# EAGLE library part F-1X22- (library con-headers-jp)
FEMALE HEADER
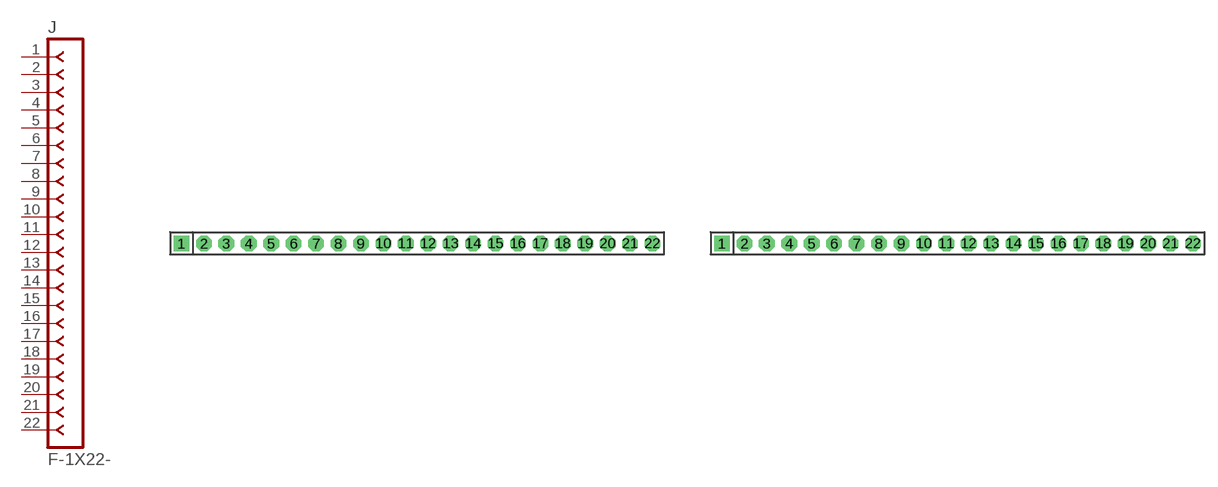
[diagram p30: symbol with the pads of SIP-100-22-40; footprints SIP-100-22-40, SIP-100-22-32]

Designator prefix J

## F-1X22-SIP-100-40  [SIP-100-22-40]
1  1  pas
2  2  pas
3  3  pas
4  4  pas
5  5  pas
6  6  pas
7  7  pas
8  8  pas
9  9  pas
10  10  pas
11  11  pas
12  12  pas
13  13  pas
14  14  pas
15  15  pas
16  16  pas
17  17  pas
18  18  pas
19  19  pas
20  20  pas
21  21  pas
22  22  pas

## F-1X22-SIP-100-32  [SIP-100-22-32]
Pads as for SIP-100-22-40

## F-1X22-SIP-100-32Y  [SIP-100-22-32Y]
Pads as for SIP-100-22-40

## F-1X22-SIP-100-40Y  [SIP-100-22-40Y]
Pads as for SIP-100-22-40

## F-1X22-KK-4455-B22  [KK-4455-B22]
Pads as for SIP-100-22-40

## F-1X22-KK-4455-C22  [KK-4455-C22]
Pads as for SIP-100-22-40

## F-1X22-KK-4455-A22  [KK-4455-A22]
Pads as for SIP-100-22-40

## Footprint SIP-100-22-40 (pad centres in mm)
SIP Header - 0.1", 40 mil drill
drill 1.016 pad 1.778 square: 1 -26.67,0
drill 1.016 pad 1.778 octagon: 2 -24.13,0; 3 -21.59,0; 4 -19.05,0; 5 -16.51,0; 6 -13.97,0; 7 -11.43,0; 8 -8.89,0; 9 -6.35,0; 10 -3.81,0; 11 -1.27,0; 12 1.27,0; 13 3.81,0; 14 6.35,0; 15 8.89,0; 16 11.43,0; 17 13.97,0; 18 16.51,0; 19 19.05,0; 20 21.59,0; 21 24.13,0; 22 26.67,0

## Footprint SIP-100-22-32 (pad centres in mm)
SIP Header - 0.1", 32 mil drill
drill 0.813 pad 1.778 square: 1 -26.67,0
drill 0.813 pad 1.778 octagon: 2 -24.13,0; 3 -21.59,0; 4 -19.05,0; 5 -16.51,0; 6 -13.97,0; 7 -11.43,0; 8 -8.89,0; 9 -6.35,0; 10 -3.81,0; 11 -1.27,0; 12 1.27,0; 13 3.81,0; 14 6.35,0; 15 8.89,0; 16 11.43,0; 17 13.97,0; 18 16.51,0; 19 19.05,0; 20 21.59,0; 21 24.13,0; 22 26.67,0

## Footprint SIP-100-22-32Y (pad centres in mm)
SIP Header - 0.1", 32 mil drill
drill 0.813 long: 1 -26.67,0; 2 -24.13,0; 3 -21.59,0; 4 -19.05,0; 5 -16.51,0; 6 -13.97,0; 7 -11.43,0; 8 -8.89,0; 9 -6.35,0; 10 -3.81,0; 11 -1.27,0; 12 1.27,0; 13 3.81,0; 14 6.35,0; 15 8.89,0; 16 11.43,0; 17 13.97,0; 18 16.51,0; 19 19.05,0; 20 21.59,0; 21 24.13,0; 22 26.67,0

## Footprint SIP-100-22-40Y (pad centres in mm)
SIP Header - 0.1", 40 mil drill
drill 1.016 long: 1 -26.67,0; 2 -24.13,0; 3 -21.59,0; 4 -19.05,0; 5 -16.51,0; 6 -13.97,0; 7 -11.43,0; 8 -8.89,0; 9 -6.35,0; 10 -3.81,0; 11 -1.27,0; 12 1.27,0; 13 3.81,0; 14 6.35,0; 15 8.89,0; 16 11.43,0; 17 13.97,0; 18 16.51,0; 19 19.05,0; 20 21.59,0; 21 24.13,0; 22 26.67,0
